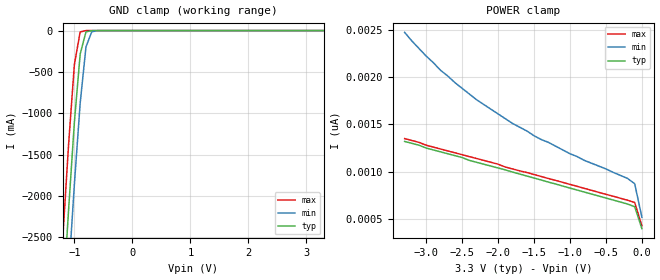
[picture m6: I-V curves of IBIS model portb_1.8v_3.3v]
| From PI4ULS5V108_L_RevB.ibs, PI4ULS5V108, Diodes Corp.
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[Model]   portb_1.8v_3.3v
Model_type Terminator
| variable   typ   min   max
C_comp   3.5237p   3.4973p   3.5489p
[Voltage Range]   3.3000V   2.9700V   3.6300V
[POWER Clamp Reference]   3.3000V   2.9700V   3.6300V
[GND Clamp Reference]   0.0000V   0.0000V   0.0000V
[Temperature Range]   25   85   -40
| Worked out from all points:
|   GND clamp passes 1 mA (typ) near -0.70 V on its own axis
[GND Clamp]
| Voltage   I(typ)   I(min)   I(max)
-3.3V     -27.9A     -28.2A     -27.6A
-1.2V     -3.31A     -4.11A     -2.51A
-1.1V     -2.17A     -2.96A     -1.38A
-1V       -1.11A     -1.86A     -411mA
-900mV    -284mA     -878mA     -15.9mA
-800mV    -15.3mA    -197mA     -233uA
-700mV    -522uA     -13.8mA    -2.03uA
-500mV    -320nA     -38.9uA    -162pA
3.3V      177pA      3.58nA     176pA
[POWER Clamp]
| Voltage   I(typ)   I(min)   I(max)
-3.3V     1.32nA     2.47nA     1.35nA
-3.2V     1.3nA      2.38nA     1.33nA
-3V       1.25nA     2.22nA     1.28nA
-2.8V     1.21nA     2.07nA     1.24nA
-2.6V     1.17nA     1.94nA     1.2nA
-2.3V     1.1nA      1.76nA     1.14nA
-1.8V     997pA      1.51nA     1.03nA
-1.5V     934pA      1.38nA     971pA
-1V       828pA      1.19nA     867pA
-200mV    660pA      930pA      700pA
-100mV    631pA      874pA      676pA
0V        400pA      520pA      429pA
